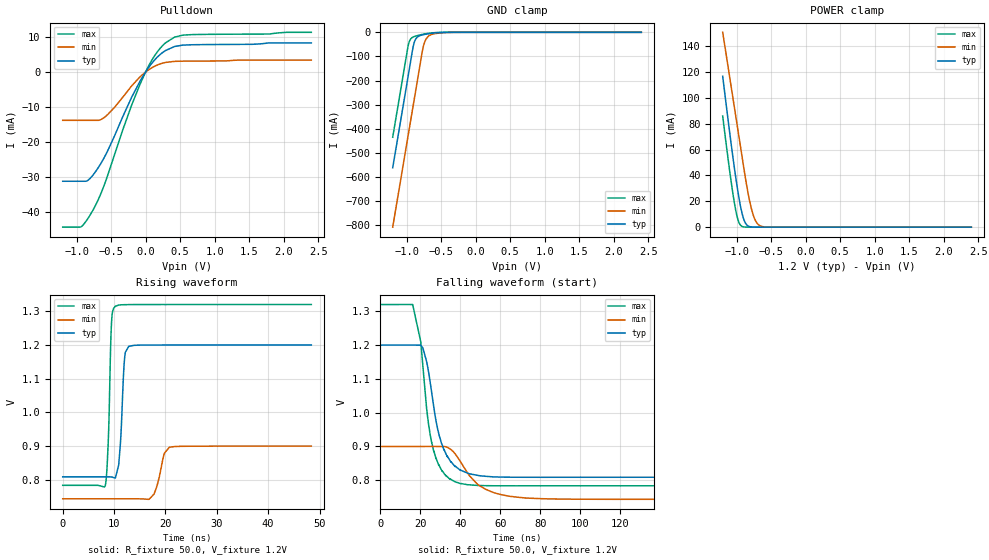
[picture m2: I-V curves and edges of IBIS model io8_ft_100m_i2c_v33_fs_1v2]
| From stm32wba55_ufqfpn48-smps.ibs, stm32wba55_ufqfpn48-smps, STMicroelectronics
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[Model]   io8_ft_100m_i2c_v33_fs_1v2
Model_type I/O_open_drain
Polarity   Non-Inverting
Enable   Active-Low
| CAP_THRESHOLD on pad IOFT is "UDTCAPC" :
| Rising=30.0% of vddiom   Falling=70.0% of vddiom
| C_comp min and max val. don't necessarily correlate with the min and max pvt
| but are the smallest and greatest pad capacitance found.
| var   typ   min   max
C_comp   1.75955pF  1.58205pF  1.89750pF
|C_comp_pulldown   1.75955pF  1.58205pF  1.89750pF
Vinl = 450.0mV
Vinh = 660.0mV
Vmeas = 600.0mV   | Reference voltage for timing measurements
Cref  = 50.0pF   | Timing specification test load capacitance value
Rref  = 1.0MOhm   | Timing specification test load resistance value
Vref  = 660.0mV   | Timing specification test load voltage
[Model Spec]
| TIME_THRESHOLD on pin ZII2CV11 is "CMOS" :
| Rising=50.0% of vdd   Falling=50.0% of vdd
Vinl 436.50000mV 342.50000mV 466.50000mV
Vinh 753.50000mV 549.50000mV 839.50000mV
| variable   typ   min   max
[Temperature Range] 25.0 140.0 -40.0
| variable   typ   min   max
[Voltage Range] 1.2V 900.0mV 1.32V
| variable   typ   min   max
[POWER Clamp Reference] 1.2V 900.0mV 1.32V
| variable   typ   min   max
[GND Clamp Reference] 0V 0V 0V
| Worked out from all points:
|   slope of the pulldown table from 0 to 0.18 V, typ, clamps not added: 40.6 ohm
|   GND clamp passes 1 mA (typ) near -0.51 V on its own axis
|   POWER clamp passes 1 mA (typ) near -0.83 V on its own axis
|   rising waveform, R_fixture 50.0, V_fixture 1.2V: 20-80 % time 747ps typ, 1.42ns min, 564ps max; typ from 0.809 V to 1.2 V
|   falling waveform, R_fixture 50.0, V_fixture 1.2V: 20-80 % time 8.05ns typ, 13.6ns min, 6.4ns max; typ from 1.2 V to 0.809 V
[POWER Clamp]
-1.2V     116.7mA    150.7mA    85.92mA
-1.06V    57.23mA    102.6mA    28.68mA
-1.02V    41.75mA    88.91mA    15.5mA
-980mV    27.6mA     75.18mA    5.935mA
-920mV    10.75mA    54.6mA     597.6uA
-870mV    3.065mA    37.68mA    60.82uA
-820mV    594.6uA    22.85mA    5.912uA
-770mV    99.71uA    11.47mA    572nA
-730mV    23.34uA    5.552mA    88.29nA
-680mV    3.779uA    1.833mA    8.565nA
-510mV    7.889nA    23.13uA    53.67pA
2.4V      0A         0A         0A
[GND Clamp]
-1.2V     -561.6mA   -807.5mA   -434.8mA
-980mV    -187.6mA   -433.5mA   -60.76mA
-960mV    -153.6mA   -399.5mA   -38.21mA
-900mV    -54.17mA   -297.5mA   -18.87mA
-870mV    -29.55mA   -246.5mA   -15.73mA
-830mV    -17.05mA   -178.5mA   -12.57mA
-760mV    -9.921mA   -62.77mA   -8.045mA
-730mV    -8.191mA   -35.56mA   -6.403mA
-680mV    -5.826mA   -15.57mA   -4.089mA
-580mV    -2.43mA    -5.043mA   -1.157mA
-330mV    -11.72uA   -245.5uA   -300.5nA
2.4V      872pA      1.056uA    338.3pA
| variable   typ   min   max
[Pullup Reference] 1.2V 900.0mV 1.32V
| variable   typ   min   max
[Pulldown Reference] 0V 0V 0V
[Pulldown]
-1.2V     -31.2mA    -13.81mA   -44.3mA
-940mV    -31.2mA    -13.81mA   -44.26mA
-850mV    -31.11mA   -13.81mA   -42.26mA
-760mV    -29.39mA   -13.81mA   -39.38mA
-660mV    -26.52mA   -13.68mA   -35.32mA
-550mV    -22.55mA   -12.17mA   -29.6mA
-330mV    -12.74mA   -7.204mA   -16.5mA
-80mV     -2.622mA   -1.37mA    -3.49mA
110mV     2.963mA    1.428mA    3.999mA
290mV     6.144mA    2.737mA    8.347mA
540mV     7.674mA    3.096mA    10.53mA
2.4V      8.312mA    3.39mA     11.33mA
[Ramp]
dV/dt_r 234.64969mV/734.00629ps 93.74533mV/1.39267ns 321.76568mV/559.54687ps
dV/dt_f 234.65882mV/7.92639ns 93.76932mV/13.23194ns 321.7731mV/6.31528ns
R_load = 50.0
| Removed startup time: 0s 0s 0s  .
| Removed end time: 48.4ns.
[Rising Waveform]
R_fixture   = 50.0
V_fixture   = 1.2V
V_fixture_min = 900.0mV
V_fixture_max = 1.32V
0s        808.9mV    743.7mV    783.7mV
8.25ns    808.9mV    743.7mV    781.3mV
8.9ns     809mV      743.7mV    926.4mV
9.5ns     808.5mV    743.7mV    1.265V
10.25ns   805.2mV    743.7mV    1.315V
11.2ns    900.8mV    743.7mV    1.319V
12.05ns   1.161V     743.7mV    1.319V
12.85ns   1.196V     743.7mV    1.32V
20.75ns   1.2V       896.6mV    1.32V
48.4ns    1.2V       900mV      1.32V
| Removed startup time: 0s 0s 0s  .
| Removed end time: 198.4ns.
[Falling Waveform]
R_fixture   = 50.0
V_fixture   = 1.2V
V_fixture_min = 900.0mV
V_fixture_max = 1.32V
0s        1.2V       900mV      1.32V
16.2ns    1.2V       900mV      1.32V
20.25ns   1.2V       900mV      1.209V
21.25ns   1.192V     900mV      1.141V
25.75ns   1.057V     900mV      909.8mV
30.6ns    909.1mV    899.9mV    830.3mV
37.4ns    842mV      878.5mV    795.3mV
48.6ns    814.6mV    788.1mV    784.7mV
64.8ns    809mV      752.5mV    783.6mV
198.4ns   808.9mV    743.7mV    783.7mV
